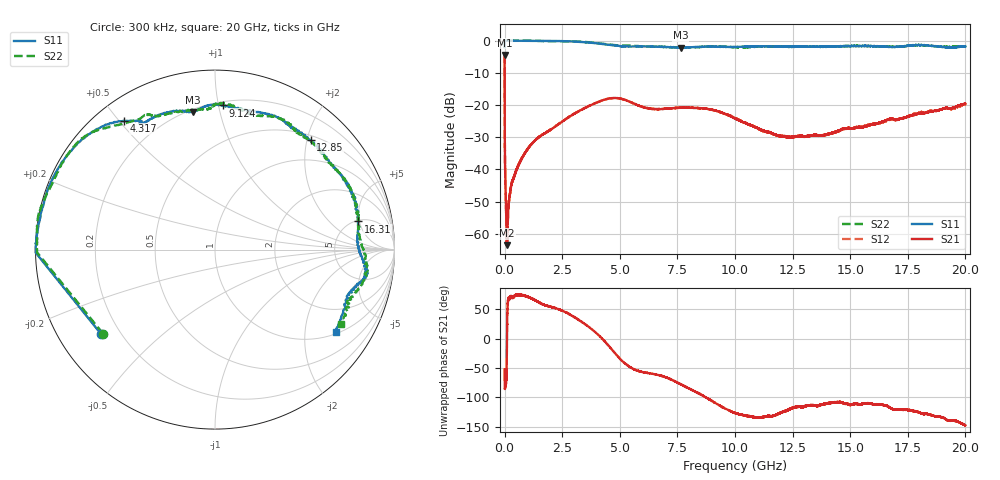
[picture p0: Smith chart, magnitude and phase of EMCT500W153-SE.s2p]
!EMCT500W153
!Johanson Technology Inc.
!www.johansontechnology.com
!Test Board Conditions:
!Substrate Type  RO4350B
!Substrate Thickness  10 mil
!Substrate Dk  3.66
!TL Type: GCPW
!TL Trace Width  22 mil
!TL Gap  14 mil
!PART MODE SINGLE ENDED (AKA BYPASS)
!DUT TOPOLOGY	SERIES-SHUNT
# MHz S  dB  R 50
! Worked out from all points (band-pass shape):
!   20001 points, 300 kHz to 20 GHz, reference 50 ohm
!   highest |S21| = -4.45 dB at 300 kHz (marker M1); lowest = -63.5 dB at 104.3 MHz (marker M2)
!   |S21| within 3 dB of the highest: start of sweep to 580.6 kHz
!   lowest |S11| = -2.2 dB at 7.639 GHz (marker M3), VSWR 7.93, Z = 10.8 + j41.5 ohm
!   |S11| at or under -10 dB: nowhere
!   |S22| runs from -2.2 to 0.0 dB; largest |S21 - S12| = 0.0055
!   S11 on the Smith chart (normalised r, x): 300 kHz: 0.13, -0.33; 4.317 GHz: 0.08, +0.51; 9.124 GHz: 0.23, +1.03; 12.85 GHz: 0.58, +2.06; 16.31 GHz: 5.17, +4.77; 20 GHz: 1.06, -2.88
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0.3  -2.05 -143.2  -4.45 -52.4  -4.43 -52.3  -2.16 -143.2
104.298  -0.01 178.8  -63.52 -1.6  -63.80 -11.2  -0.08 179.1
163.298  0.00 178.0  -52.49 67.2  -52.19 68.3  -0.08 178.4
280.296  -0.03 176.8  -45.21 72.1  -45.16 71.4  -0.06 176.8
488.293  -0.05 174.5  -40.74 74.7  -40.73 73.5  -0.04 174.4
1061.284  -0.08 167.8  -33.01 70.5  -33.05 70.4  -0.01 167.3
2214.267  -0.12 154.5  -26.60 51.9  -26.54 51.6  -0.19 153.1
3334.25  -0.44 137.0  -21.47 28.9  -21.48 28.8  -0.34 138.8
4317.235  -1.12 125.4  -18.38 -3.5  -18.36 -3.6  -1.04 128.8
5100.224  -1.77 120.5  -18.11 -37.9  -18.15 -37.9  -1.49 117.4
6667.2  -1.89 106.7  -21.30 -62.0  -21.26 -62.3  -1.93 109.1
7639.185  -2.20 99.0  -20.85 -77.9  -20.86 -77.7  -2.10 97.2
9124.163  -1.89 87.0  -21.68 -109.2  -21.72 -108.9  -1.78 87.7
10000.15  -1.99 76.7  -24.15 -126.8  -24.02 -126.7  -2.12 77.8
11770.12  -1.86 59.6  -29.30 -130.0  -29.29 -129.0  -1.78 58.8
12848.11  -1.83 48.9  -29.53 -115.9  -29.43 -116.2  -1.92 50.1
13334.1  -1.90 42.0  -29.46 -113.7  -29.46 -114.1  -1.92 44.0
16307.06  -1.80 11.1  -25.41 -112.5  -25.57 -113.5  -1.73 11.3
16667.05  -1.95 5.6  -24.41 -116.5  -24.68 -116.2  -1.86 8.0
18031.03  -1.45 -9.6  -22.57 -126.4  -22.36 -126.8  -1.46 -9.0
19291.01  -2.11 -20.0  -21.00 -139.9  -21.22 -141.8  -2.01 -21.7
20000  -1.80 -34.3  -19.56 -148.1  -19.79 -145.9  -1.76 -30.7
